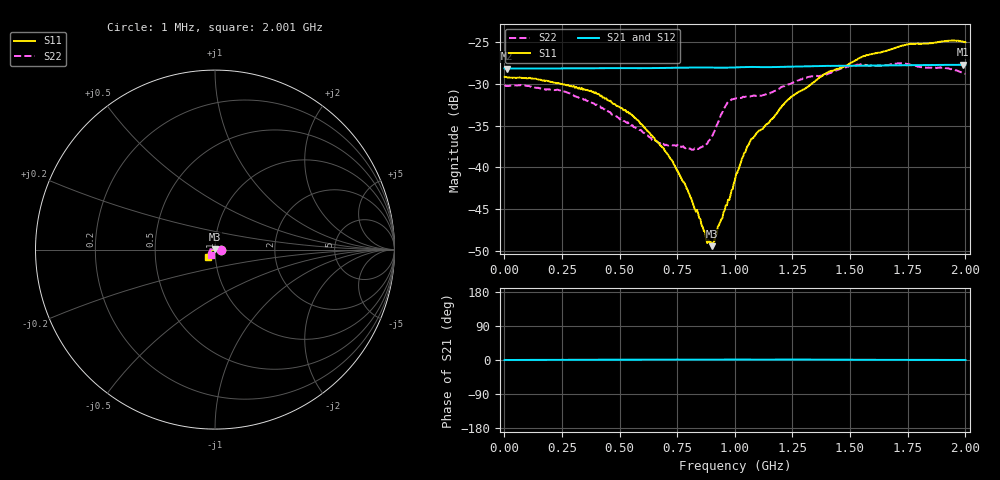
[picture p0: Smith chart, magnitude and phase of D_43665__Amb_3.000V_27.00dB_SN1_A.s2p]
! device id: 43665_
! dir: \\malibu\benchdata\1_engineers\tn_data\43665_75ohm\new\sparar\43665_\amb\3p000v\27p00db
! Serial: 1
! Insertion: A
! Temp: Amb
! VDD: 3.000V
! Attenuation Step: 27.00dB
! IDD: 1.450884e+00mA
! FILE NAME
! DATE 03-27-2009 08:40:01
! CORRECTED  DATA
#  Hz  S  RI  R  75
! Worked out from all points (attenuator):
!   401 points, 1 MHz to 2.001 GHz, reference 75 ohm
!   highest |S21| = -27.71 dB at 1.991 GHz (marker M1); lowest = -28.2 dB at 11 MHz (marker M2)
!   lowest |S11| = -49.4 dB at 901 MHz (marker M3), VSWR 1.01, Z = 74.7 + j0.378 ohm
!   |S11| at or under -10 dB: start of sweep to end of sweep
!   |S22| runs from -37.9 to -27.5 dB; largest |S21 - S12| = 0.00048
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1000000  0.0349 -0.000394  0.0392 -0.000133  0.0393 -7.18e-05  0.0311 -0.000169
1.1e7  0.0347 0.000152  0.0391 -2.77e-05  0.0391 -8.38e-06  0.0308 0.00017
2.36e8  0.0317 0.00427  0.0391 0.000323  0.0392 0.000337  0.027 0.0107
3.36e8  0.0294 0.00547  0.0392 0.000414  0.0392 0.000484  0.0217 0.014
5.46e8  0.0198 0.00725  0.0393 0.000546  0.0393 0.000443  0.00893 0.0159
6.71e8  0.0125 0.00632  0.0394 0.000736  0.0394 0.000635  0.000684 0.014
7.31e8  0.00899 0.00601  0.0395 0.000714  0.0395 0.000627  -0.00339 0.0131
8.21e8  0.00359 0.00471  0.0396 0.000711  0.0396 0.000552  -0.00964 0.00836
8.76e8  -0.000311 0.00371  0.0396 0.000646  0.0396 0.000506  -0.013 0.0043
9.01e8  -0.00224 0.00253  0.0396 0.000613  0.0396 0.000505  -0.0151 0.00245
9.11e8  -0.00297 0.00206  0.0396 0.00064  0.0396 0.000464  -0.0163 0.00169
9.61e8  -0.00585 0.000891  0.0395 0.000768  0.0396 0.000612  -0.0235 0.000977
1.001e9  -0.00844 0.000397  0.0397 0.000914  0.0397 0.000754  -0.0257 0.00236
1.041e9  -0.0122 -0.000688  0.0399 0.00088  0.0399 0.000698  -0.0264 0.000928
1.081e9  -0.0148 -0.00256  0.0399 0.000629  0.04 0.000503  -0.0269 -0.00185
1.231e9  -0.024 -0.00861  0.04 0.000824  0.0401 0.000602  -0.0296 -0.0104
1.336e9  -0.0287 -0.0138  0.0404 0.000733  0.0405 0.000582  -0.0313 -0.0159
1.551e9  -0.0378 -0.0258  0.0406 0.000434  0.0407 0.000142  -0.0319 -0.0261
1.671e9  -0.0396 -0.0313  0.0408 0.000301  0.0409 -1.03e-05  -0.0304 -0.0278
1.756e9  -0.0407 -0.0366  0.0409 0.000229  0.041 -9.64e-05  -0.0283 -0.0303
1.991e9  -0.0373 -0.0426  0.0412 9.73e-05  0.0413 -0.000325  -0.0229 -0.0288
2.001e9  -0.037 -0.0422  0.0411 0.000106  0.0412 -0.000335  -0.0226 -0.0284
